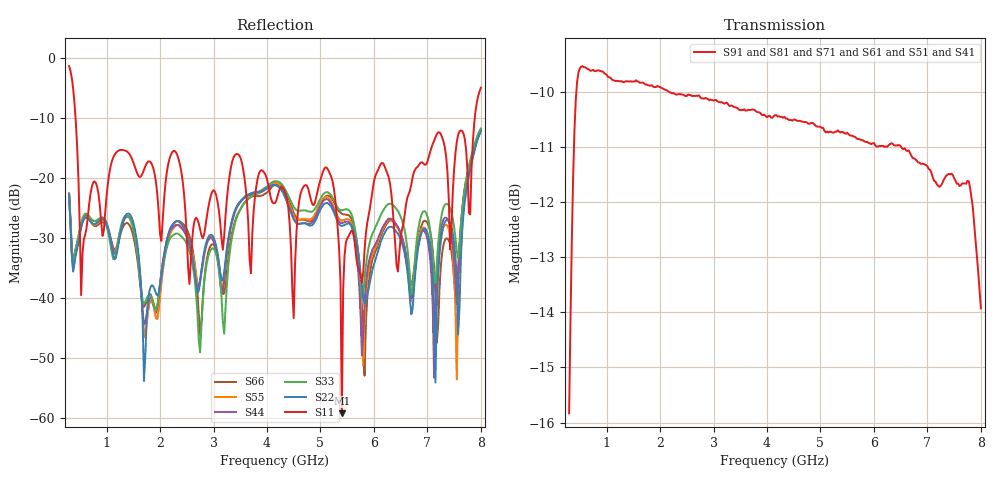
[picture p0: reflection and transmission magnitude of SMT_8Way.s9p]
! Created Thu Nov 23 10:06:52 2017
# hz S ma R 50
! 9 Port Network Data from SP1.SP block
! freq  magS11  angS11  magS12  angS12  magS13  angS13  magS14  angS14
!  magS15  angS15  magS16  angS16  magS17  angS17  magS18  angS18
!  magS19  angS19
!  magS21  angS21  magS22  angS22  magS23  angS23
!  magS24  angS24  magS25  angS25  magS26  angS26  magS27  angS27
!  magS28  angS28  magS29  angS29
!  magS31  angS31  magS32  angS32
!  magS33  angS33  magS34  angS34  magS35  angS35  magS36  angS36
!  magS37  angS37  magS38  angS38  magS39  angS39
!  magS41  angS41
!  magS42  angS42  magS43  angS43  magS44  angS44  magS45  angS45
!  magS46  angS46  magS47  angS47  magS48  angS48  magS49  angS49
!  magS51  angS51  magS52  angS52  magS53  angS53  magS54  angS54
!  magS55  angS55  magS56  angS56  magS57  angS57  magS58  angS58
!  magS59  angS59
!  magS61  angS61  magS62  angS62  magS63  angS63
!  magS64  angS64  magS65  angS65  magS66  angS66  magS67  angS67
!  magS68  angS68  magS69  angS69
!  magS71  angS71  magS72  angS72
!  magS73  angS73  magS74  angS74  magS75  angS75  magS76  angS76
!  magS77  angS77  magS78  angS78  magS79  angS79
!  magS81  angS81
!  magS82  angS82  magS83  angS83  magS84  angS84  magS85  angS85
!  magS86  angS86  magS87  angS87  magS88  angS88  magS89  angS89
!  magS91  angS91  magS92  angS92  magS93  angS93  magS94  angS94
!  magS95  angS95  magS96  angS96  magS97  angS97  magS98  angS98
!  magS99  angS99
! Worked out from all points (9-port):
!   309 points, 300 MHz to 8 GHz, reference 50 ohm
!   strongest paths, dB at 300 MHz, 2.225 GHz, 4.15 GHz, 6.075 GHz, 8 GHz:
!     S91: -15.8, -10.0, -10.4, -11.0, -13.9
!     S81: -15.9, -10.0, -10.4, -11.0, -14.0
!     S71: -15.9, -10.1, -10.5, -11.1, -14.1
!     S61: -15.9, -10.1, -10.6, -11.1, -14.0
!     S51: -16.0, -10.1, -10.6, -11.1, -14.0
!     S41: -15.9, -10.1, -10.6, -11.2, -14.1
!   lowest |S11| = -59.3 dB at 5.4 GHz (marker M1), VSWR 1.00, Z = 50 - j0.104 ohm
!   |S11| at or under -10 dB: 419.9 MHz to 7.886 GHz (7.466 GHz wide, 180 % of centre)
